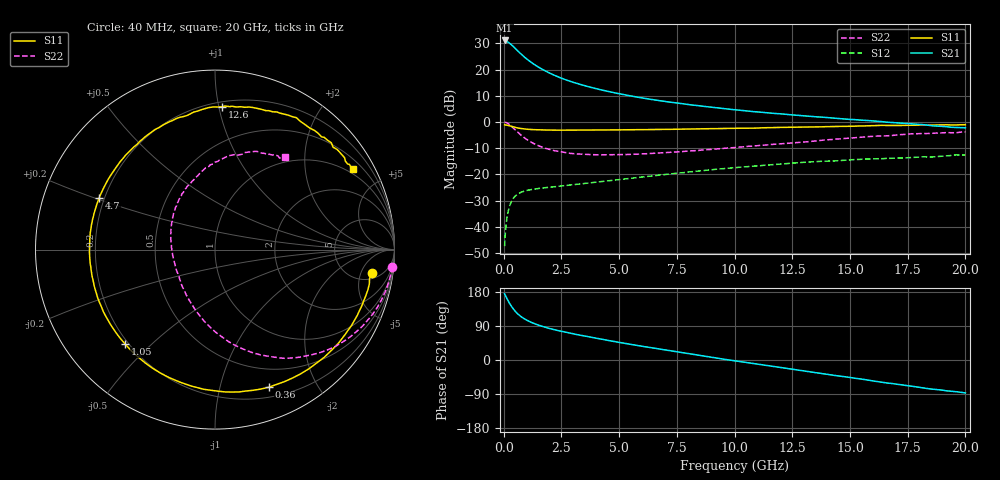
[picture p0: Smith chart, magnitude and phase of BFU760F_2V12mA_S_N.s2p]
! Filename:  P:\Prog\Test\Noise\ATS_data\Testdata_Net\BFU760\BFU760F_2W_C1_2V12mA_D.s2p
! Date/Time: Mon 06/Feb/2012 15:05:25
! BFU760_2W_C1_2V12mA
! bias mode 1: Vout= 2.0002 V, Iout=11.9300 mA, Vin= 0.7772 V, Iin= 0.0355 mA
! Date/time Fri Mar 18 13:30:22 2011
! Device data file deembeded for feedlines and parallel
! Original file: \BFU760\BFU760_2W_C1_2V12mA_R.s2p
! Feed-files: PR003V01_101208_Feed1.s2p, PR003V01_101208_Feed2.s2p
! Parallel-file: PR003V01_101208_Par.s2p
# MHz S MA R 50
!  Freq-MHz  S11-mag  S11-arg  S21-mag  S21-arg  S12-mag  S12-arg  S22-mag  S22-arg
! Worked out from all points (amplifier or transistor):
!   167 points, 40 MHz to 20 GHz, reference 50 ohm
!   highest |S21| = 31.1 dB at 40 MHz (marker M1)
!   |S21| within 3 dB of that: start of sweep to 497.1 MHz
!   unconditionally stable (mu >= 1): 4.993 GHz to 13.55 GHz
!   at 550 MHz: K = 0.15, MSG = 27.8 dB, |S12| = -27.9 dB
!   at 4.2 GHz: K = 0.92, MSG = 17.5 dB, |S12| = -22.8 dB
!   at 20 GHz: K = 0.85, MSG = 5.2 dB, |S12| = -12.6 dB
!   lowest NFmin = 0.45 dB at 400 MHz
!   S11 on the Smith chart (normalised r, x): 40 MHz: 7, -8; 360 MHz: 0.30, -1.42; 1.05 GHz: 0.19, -0.42; 4.7 GHz: 0.18, +0.21; 12.6 GHz: 0.23, +1.02; 20 GHz: 0.83, +3.52
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40  0.8829 -8.5  35.89 174.9  0.004294 83.8  0.9912 -5.5
50  0.8759 -10.7  35.86 173.1  0.00538 78.5  0.9895 -7.0
120  0.8731 -25.1  34.87 164.6  0.01266 77.0  0.969 -16.8
220  0.8544 -44.7  32.77 153.1  0.02199 67.6  0.912 -29.9
280  0.8405 -55.5  31.19 146.9  0.02673 62.5  0.871 -37.0
360  0.823 -68.7  29.02 139.6  0.03192 56.4  0.8081 -45.8
460  0.7987 -83.4  26.44 131.4  0.03708 50.1  0.7358 -55.2
550  0.781 -94.5  24.15 125.2  0.04039 45.6  0.6713 -62.6
650  0.7638 -104.8  21.8 119.5  0.04338 41.5  0.6132 -69.8
850  0.7417 -121.4  18.05 110.4  0.04745 35.7  0.5186 -81.6
1050  0.7262 -133.6  15.27 103.5  0.05004 32.1  0.4494 -91.1
1400  0.7127 -148.9  11.9 94.4  0.05321 28.5  0.3704 -104.6
1850  0.7034 -162.2  9.186 85.5  0.05626 26.4  0.3115 -118.4
2500  0.6998 -175.5  6.854 75.7  0.06025 25.7  0.2687 -134.5
3400  0.7008 171.1  5.083 64.4  0.06656 25.5  0.2438 -151.2
4700  0.7069 155.8  3.685 49.7  0.07725 25.2  0.2375 -171.4
6800  0.7215 135.3  2.538 28.4  0.09774 21.6  0.2574 163.2
10200  0.7613 106.5  1.682 -3.9  0.1368 8.5  0.333 129.2
12600  0.7965 87.3  1.354 -25.2  0.1654 -4.1  0.402 108.3
13400  0.8032 81.5  1.27 -32.1  0.1745 -9.5  0.4307 101.7
16800  0.8584 55.1  0.9773 -61.9  0.2036 -30.4  0.5531 74.0
20000  0.8883 30.2  0.7749 -87.0  0.2349 -52.2  0.6487 52.8
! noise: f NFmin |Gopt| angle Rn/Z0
400  0.4458  0.1083  4.9  0.0621
700  0.4485  0.1079  51.99  0.0601
1200  0.4581  0.1729  92.62  0.0566
1600  0.4704  0.2233  108.4  0.0536
2000  0.4867  0.2639  120.6  0.0506
2400  0.507  0.2975  131.8  0.0476
3100  0.5524  0.3515  150.6  0.0426
3900  0.6194  0.4217  169.8  0.0375
4700  0.7025  0.5004  185  0.0335
6000  0.8723  0.5897  200.7  0.0305
